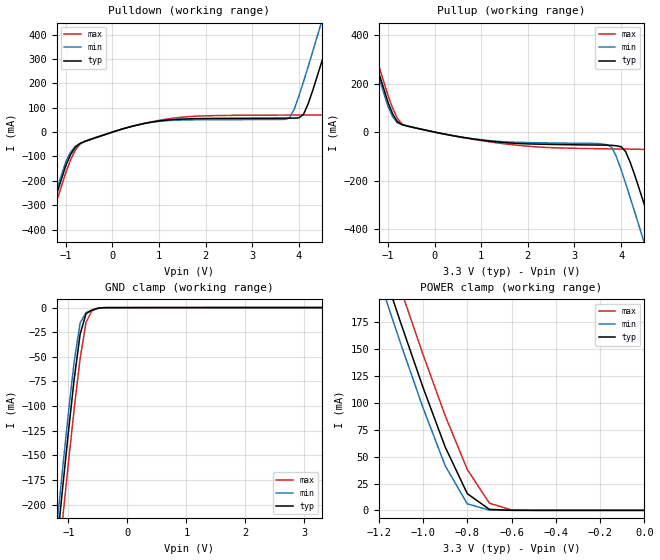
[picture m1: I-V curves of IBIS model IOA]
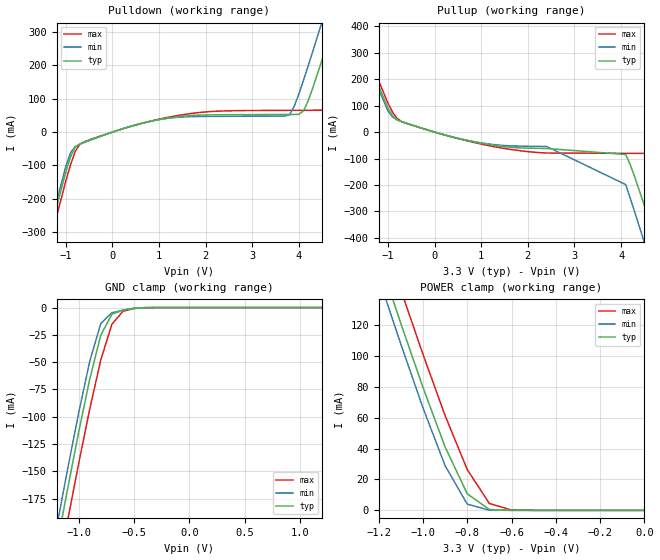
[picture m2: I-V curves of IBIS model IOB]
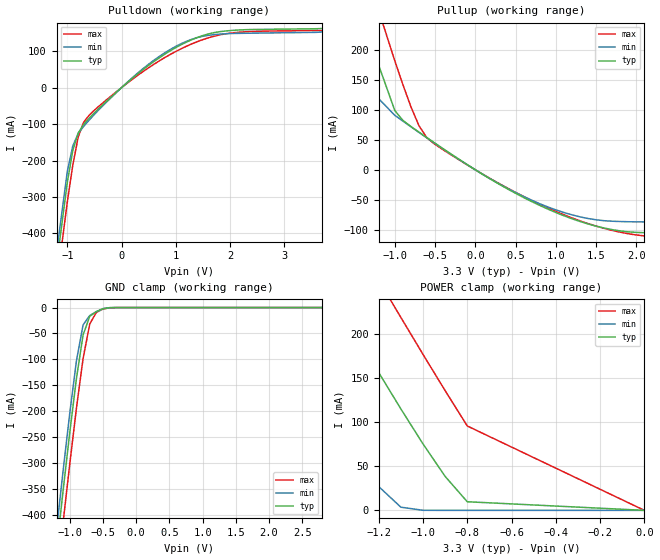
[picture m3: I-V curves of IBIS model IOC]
| IBIS file Qspan.ibs created by s2ibis2 version 2.1
[IBIS ver]   2.1
[File name]   qspn2a3.ibs
[File Rev]   1.0
[Date]   03- 03- 2000
[Notes]   The data is simulation based
|   This is for modelling purposes only.
|   History : #3591862.MI001.01 - Pin List corrections.
|   #3591862.MI001.02 - Revised Power Pins.
|   #3591862.MI001.03 - Updated with IDT formtting
|   This is the Qspan II (CA91L862A-XXE, 27mm PBGA) IBIS
|   MODEL for a 3.3 V PCI signalling environment.
[Disclaimer] This model is subject to change.
   Integrated Device Technology, Inc. ("IDT") hereby grants the
   user of this IBIS model a non-exclusive, nontransferable
   license to use this IBIS model under the following terms. The
   user is granted this license only to use the IBIS model and is
   not granted rights to sell, copy (except as needed to run the
   IBIS model), rent, lease or sub-license the IBIS model in
   whole or in part, or in modified form to anyone. The User may
   modify the IBIS model to suit its specific applications, but
   rights to derivative works and such modifications shall belong
   to IDT. This IBIS model is provided on an AS IS" basis and IDT
   makes absolutely no warranty with respect to the information
   contained herein. IDT DISCLAIMS AND CUSTOMER WAIVES ALL
   WARRANTIES, EXPRESS AND IMPLIED, INCLUDING WARRANTIES OF
   MERCHANTABILITY AND FITNESS FOR A PARTICULAR PURPOSE. THE
   ENTIRE RISK AS TO QUALITY AND PERFORMANCE IS WITH THE USER
   ACCORDINGLY, IN NO EVENT SHALL IDT BE LIABLE FOR ANY DIRECT OR
   INDIRECT DAMAGES, WHETHER IN CONTRACT OR TORT, INCLUDING ANY
   LOST PROFITS OR OTHER INCIDENTAL, CONSEQUENTIAL, EXEMPLARY, OR
   PUNITIVE DAMAGES ARISING OUT OF THE USE OR APPLICATION OF THE
   IBIS model. Further, IDT reserves the right to make changes
   without notice to any product herein to improve reliability,
   function, or design. IDT does not convey any license under
   patent rights or any other intellectual property rights,
   including those of third parties. IDT is not obligated to
   provide maintenance or support for the licensed IBIS model.
[Copyright]   Copyright 2009, Integrated Device Technology, Inc. all
   rights reserved.
|   Component QSPAN
[Component]   QSPAN
[Manufacturer]   Integrated Device Technology, Inc.
[Package]
| variable   typ   min   max
R_pkg   45m   22m   75m
L_pkg   2.5nH   1.1nH   4.3nH
C_pkg   1.3pF   1.2pF   1.4pF
[Pin]  signal_name   model_name
 A2   D26   IOA
 C2   D27   IOA
 B1   D28   IOA
 D3   D29   IOA
 C1   D30   IOA
 E4   D31   IOA
 E3   A26   IOA
 E1   A27   IOA
 F2   A28   IOA
 G2   A29   IOA
 H3   A30   IOA
 H2   A31   IOA
 G3   R/W   IOA
 H1   DSACK1/TA   IOB
 J4   DSACK0   IOB
 J3   SIZ1   IOA
 J2   SIZ0   IOA
 J1   SDA   IOB
 K3   SCL   OUTA
 L1   IMSEL   INA
 W19   VSS   GND
 L3   TMODE1   IOD
 M1   TMODE0   IOD
 M3   RESETI   INB
 N1   RESETO   IOF
 N3   BURST/TIP   IOA
 P2   TS   IOB
 R1   BB/BGACK   IOB
 R2   BR   OUTA
 T3   REQ   IOC
 T4   AD31   IOC
 V2   AD30   IOC
 U3   AD29   IOC
 W1   AD28   IOC
 W2   AD27   IOC
 T1   HALT/RETRY   IOB
 U2   GNT   IOC
 P4   RST   INC
 W11   PCLK   INC
 M20   BM_EN   IOD
 Y1   AD26   IOC
 Y2   AD25   IOC
 W3   AD24   IOC
 W4   C/BE3   IOC
 U5   AD23   IOC
 V7   AD22   IOC
 Y7   AD21   IOC
 V8   AD20   IOC
 W8   AD19   IOC
 Y8   AD18   IOC
 U9   AD17   IOC
 W9   AD16   IOC
 Y9   C/BE2   IOC
 W10   FRAME   IOC
 V10   IRDY   IOC
 Y10   TRDY   IOC
 Y11   DEVSEL   IOC
 V11   STOP   IOC
 U11   PERR   IOC
 Y12   PAR   IOC
 W12   C/BE1   IOC
 V12   AD15   IOC
 Y13   AD14   IOC
 W13   AD13   IOC
 V13   AD12   IOC
 Y14   AD11   IOC
 W14   AD10   IOC
 Y15   AD9   IOC
 V14   AD8   IOC
 W15   C/BE0   IOC
 Y16   IDSEL   INC
 U14   AD7   IOC
 W18   AD6   IOC
 V18   AD5   IOC
 Y20   AD4   IOC
 V19   AD3   IOC
 W20   AD2   IOC
 U18   AD1   IOC
 V20   AD0   IOC
 T19   CSREG   INA
 R20   CSPCI   INA
 P18   TC0   IOA
 P19   TC1   IOA
 P20   TC2   IOA
 N18   TC3   IOA
 N19   BERR/TEA   IOB
 N20   AS   IOB
 M17   BDIP   IOA
 M18   BG   INA
 J18   ENID   IOD
 K19   DACK/SDACK   INB
 K17   DONE   INA
 J19   QINT   IOE
 J17   DREQ   OUTA
 T18   INT   IOC
 U20   SERR   IOC
 G20   A0   IOA
 G19   A1   IOA
 F20   A2   IOA
 F19   A3   IOA
 E20   A4   IOA
 G17   A5   IOA
 F18   D0   IOA
 E19   D1   IOA
 E18   D2   IOA
 E17   D3   IOA
 C20   D4   IOA
 D18   D5   IOA
 P3   VSS   GND
 A10   QCLK   INA
 L20   VSS   GND
 A8   VSS   GND
 B20   D6   IOA
 B19   D7   IOA
 C18   D8   IOA
 A20   D9   IOA
 B18   D10   IOA
 A19   D11   IOA
 C17   A6   IOA
 B17   A7   IOA
 A18   A8   IOA
 B16   A9   IOA
 C16   A10   IOA
 C14   A11   IOA
 B14   A12   IOA
 A14   A13   IOA
 C13   A14   IOA
 B13   A15   IOA
 A13   DS   OUTA
 D12   D12   IOA
 C12   D13   IOA
 B12   D14   IOA
 B11   D15   IOA
 C11   D16   IOA
 A11   D17   IOA
 B10   D18   IOA
 C10   D19   IOA
 D10   A16   IOA
 A9   A17   IOA
 C9   A18   IOA
 D9   A19   IOA
 B8   A20   IOA
 C8   A21   IOA
 A7   A22   IOA
 B7   A23   IOA
 A6   A24   IOA
 C7   A25   IOA
 B6   D20   IOA
 D7   D21   IOA
 A3   D22   IOA
 C4   D23   IOA
 D5   D24   IOA
 B3   D25   IOA
 J20   TCK   INF
 L18   TDI   INF
 M19   TDO   OUTA
 K20   TMS   INF
 K18   TRST   INF
 K1   ENUM   IOF
 N2   HS_HEALTHY   IOD
 L2   HS_LED   IOF
 L4   HS_SWITCH   IOD
 M4   PCI_DIS   IOD
 M2   PME   IOF
 C5   DP3   IOA
 A4   DP2   IOA
 B5   DP1   IOA
 C6   DP0   IOA
 B4   PCI_ARB_EN   IOD
 B15   BIDIR_CTRL/Test1 ING
 D14   RAM_WE/TEST2   IOD
 C15   TMODE[2]/Test3 IOD
 V5   EXT_GNT[1]   OUTB
 W5   EXT_GNT[2]   OUTB
 Y5   EXT_GNT[3]   OUTB
 V6   EXT_GNT[4]   OUTB
 U7   EXT_GNT[5]   OUTB
 W6   EXT_GNT[6]   OUTB
 Y17   EXT_REQ[1]   IOC
 V16   EXT_REQ[2]   IOC
 W17   EXT_REQ[3]   IOC
 Y18   EXT_REQ[4]   IOC
 U16   EXT_REQ[5]   IOC
 V17   EXT_REQ[6]   IOC
 R3   VH   POWER
 D1   VSS   GND
 F1   VSS   GND
 D2   VDD   POWER
 U1   VSS   GND
 T2   VDD   POWER
 V1   VSS   GND
 V3   VDD   POWER
 W7   VSS   GND
 V9   VSS   GND
 U12   VDD   POWER
 Y19   VDD   POWER
 U19   VDD   POWER
 T17   VSS   GND
 H19   VSS   GND
 G18   VDD   POWER
 D20   VDD   POWER
 D19   VSS   GND
 C19   VDD   POWER
 D16   VDD   POWER
 A12   VSS   GND
 D6   VDD   POWER
 D11   VDD   POWER
 D15   VDD   POWER
 F4   VDD   POWER
 F17   VDD   POWER
 K4   VDD   POWER
 L17   VDD   POWER
 R4   VDD   POWER
 R17   VDD   POWER
 U6   VDD   POWER
 U10   VDD   POWER
 U15   VDD   POWER
 A5   VDD   POWER
 E2   VDD   POWER
 B2   VDD   POWER
 A1   VSS   GND
 D4   VSS   GND
 D8   VSS   GND
 D13   VSS   GND
 D17   VSS   GND
 H4   VSS   GND
 H17   VSS   GND
 N4   VSS   GND
 N17   VSS   GND
 U4   VSS   GND
 U8   VSS   GND
 U13   VSS   GND
 U17   VSS   GND
| Models and submodels in the file (14): IOA (I/O), IOB (I/O), IOC (I/O), IOD (I/O), IOE (I/O), IOF (I/O), INA (Input), INB (Input), INC (Input), IND (Input), INF (Input), ING (Input), OUTA (Output), OUTB (Output)
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|   Model IOA
[Model]   IOA
Model_type   I/O
Polarity   Non-Inverting
Vinl =   0.8000V
Vinh =   2.0000V
C_comp   5.00pF   5.00pF   5.00pF
[Voltage Range]   3.3000V   3.0000V   4.0000V
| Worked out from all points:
|   slope of the pulldown table from 0 to 0.495 V, typ, clamps not added: 18.2 ohm
|   slope of the pullup table from 0 to 0.495 V, typ, clamps not added: 27.2 ohm
|   GND clamp passes 1 mA (typ) near -0.52 V on its own axis
|   POWER clamp passes 1 mA (typ) near -0.70 V on its own axis
[Pulldown]
| voltage   I(typ)   I(min)   I(max)
-3.3V     -1.576A    -1.558A    -1.604A
-1.5V     -432.5mA   -413.1mA   -463.7mA
-1V       -137.3mA   -121.2mA   -166mA
-800mV    -62.87mA   -58.79mA   -74.96mA
-500mV    -31.87mA   -32.96mA   -30.93mA
1V        45.56mA    44.16mA    48.21mA
3.7V      57.2mA     52.22mA    69.71mA
4V        58.41mA    148mA      69.9mA
4.5V      294.4mA    461.1mA    70.42mA
4.7V      421.5mA    591.5mA    77.39mA
5.3V      814mA      988.5mA    402.9mA
6.6V      1.688A     1.867A     1.263A
[Pullup]
| voltage   I(typ)   I(min)   I(max)
-3.3V     1.609A     1.592A     1.638A
-1.7V     557.5mA    538.6mA    588mA
-1.5V     428.5mA    409.4mA    459.4mA
-1V       122.4mA    105.5mA    151.3mA
-700mV    30.44mA    30.51mA    33.57mA
1.3V      -39.66mA   -37.29mA   -43.6mA
3.8V      -54.6mA    -62.87mA   -69.47mA
4.1V      -81.22mA   -213.1mA   -70.13mA
4.5V      -300mA     -458.7mA   -71.63mA
4.7V      -422.9mA   -584.6mA   -86.04mA
5.3V      -800.7mA   -966.3mA   -409.6mA
6.6V      -1.632A    -1.801A    -1.229A
[GND_clamp]
| voltage   I(typ)   I(min)   I(max)
-3.3V     -1.575A    -1.558A    -1.603A
-1.2V     -245.1mA   -225.4mA   -276.9mA
-1.1V     -185.2mA   -165.4mA   -216.9mA
-1V       -127mA     -107.6mA   -158.4mA
-900mV    -72.3mA    -54.37mA   -102.3mA
-800mV    -26.9mA    -15.62mA   -51.61mA
-700mV    -6.214mA   -5.156mA   -14.97mA
-600mV    -2.552mA   -2.501mA   -3.238mA
-500mV    -695.8uA   -617.9uA   -852uA
-400mV    -107.6uA   -78.58uA   -172.5uA
3.3V      28.55pA    37.85pA    -1.579uA
[POWER_clamp]
| voltage   I(typ)   I(min)   I(max)
-3.3V     1.609A     1.591A     1.638A
-1.2V     236mA      216.5mA    267.2mA
-1.1V     174.3mA    154.8mA    205.5mA
-1V       114.6mA    95.56mA    145.3mA
-900mV    59.17mA    41.7mA     88.32mA
-800mV    15.58mA    6.074mA    38.1mA
-700mV    917.4uA    198.5uA    6.641mA
-600mV    41.48uA    8.933uA    391uA
0V        28.55pA    15.28pA    402.7pA
[Ramp]
| variable   typ   min   max
dV/dt_r   1.1938/1.0833n   1.0738/1.1037n   1.4781/1.0201n
dV/dt_f   1.3746/0.6576n   1.2583/0.6707n   1.6602/0.6545n
R_load = 50.0000
| End [Model] IOA
|   Model IOB
[Model]   IOB
Model_type   I/O
Polarity   Non-Inverting
Vinl =   0.8000V
Vinh =   2.0000V
C_comp   5.00pF   5.00pF   5.00pF
[Voltage Range]   3.3000V   3.0000V   4.0000V
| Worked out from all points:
|   slope of the pulldown table from 0 to 0.495 V, typ, clamps not added: 23.4 ohm
|   slope of the pullup table from 0 to 0.495 V, typ, clamps not added: 21.1 ohm
|   GND clamp passes 1 mA (typ) near -0.52 V on its own axis
|   POWER clamp passes 1 mA (typ) near -0.70 V on its own axis
[Pulldown]
| voltage   I(typ)   I(min)   I(max)
-3.3V     -1.412A    -1.395A    -1.438A
-1.5V     -386.4mA   -368.6mA   -415.1mA
-900mV    -74.1mA    -62.08mA   -98.15mA
-700mV    -35.4mA    -36.6mA    -36.59mA
-500mV    -24.52mA   -25.57mA   -23.57mA
1.3V      44.42mA    43.02mA    47.13mA
3.8V      52.72mA    51.97mA    65.13mA
4.1V      63.59mA    155.8mA    65.28mA
4.5V      217.2mA    331.9mA    65.51mA
4.7V      305.5mA    422.4mA    70.09mA
5.3V      577.8mA    698mA      295.9mA
6.6V      1.186A     1.309A     892.4mA
[Pullup]
| voltage   I(typ)   I(min)   I(max)
-3.3V     1.118A     1.106A     1.138A
-1.9V     478.2mA    465.2mA    499.2mA
-1.7V     388mA      374.9mA    409.2mA
-1V       89.64mA    79.2mA     108.7mA
-600mV    32.82mA    33.32mA    32.7mA
1V        -42.36mA   -40.74mA   -45.36mA
2.4V      -61.9mA    -54.17mA   -79.11mA
4.1V      -84.69mA   -198.5mA   -80.23mA
4.5V      -278mA     -416.8mA   -80.51mA
4.7V      -387.4mA   -528.9mA   -94.37mA
5.3V      -724.1mA   -869.2mA   -380.8mA
6.6V      -1.467A    -1.615A    -1.112A
[GND_clamp]
| voltage   I(typ)   I(min)   I(max)
-3.3V     -1.411A    -1.395A    -1.438A
-1.2V     -219.7mA   -201.6mA   -248.8mA
-1.1V     -166.1mA   -148mA     -195.1mA
-1V       -114.1mA   -96.4mA    -142.8mA
-900mV    -65.46mA   -49.1mA    -92.83mA
-800mV    -25.26mA   -14.59mA   -47.88mA
-700mV    -6.072mA   -4.689mA   -15.35mA
-600mV    -2.394mA   -2.36mA    -3.375mA
-500mV    -685.3uA   -610.9uA   -846.3uA
-400mV    -76.55uA   -48.08uA   -135.9uA
1.2V      4.332pA    -1.927pA   212.7pA
[POWER_clamp]
| voltage   I(typ)   I(min)   I(max)
-3.3V     1.117A     1.105A     1.137A
-1.2V     163.9mA    150.4mA    185.6mA
-1.1V     121mA      107.6mA    142.7mA
-1V       79.56mA    66.32mA    101mA
-900mV    41.02mA    28.91mA    61.3mA
-800mV    10.7mA     4.026mA    26.39mA
-700mV    530.2uA    85.3uA     4.443mA
-600mV    12.01uA    1.252uA    210.9uA
0V        46.55pA    30.21pA    403.7pA
[Ramp]
| variable   typ   min   max
dV/dt_r   1.3368/0.5001n   1.2090/0.4937n   1.6416/0.4419n
dV/dt_f   1.2654/0.2879n   1.1628/0.2678n   1.5276/0.2973n
R_load = 50.0000
| End [Model] IOB
|   Model IOC
[Model]   IOC
Model_type   I/O
Polarity   Non-Inverting
Vinl =   0.8000V
Vinh =   2.0000V
C_comp   5.00pF   5.00pF   5.00pF
[Voltage Range]   3.3000V   3.0000V   3.5000V
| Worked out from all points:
|   slope of the pulldown table from 0 to 0.495 V, typ, clamps not added: 8.19 ohm
|   slope of the pullup table from 0 to 0.495 V, typ, clamps not added: 12.7 ohm
|   GND clamp passes 1 mA (typ) near -0.44 V on its own axis
[Pulldown]
| voltage   I(typ)   I(min)   I(max)
-3.3V     -3.036A    -3.001A    -3.093A
-1.5V     -828mA     -790.5mA   -888.2mA
-1V       -258.8mA   -229mA     -312.4mA
-900mV    -172.7mA   -160.1mA   -212.7mA
-800mV    -124.4mA   -125.9mA   -135.4mA
-700mV    -100.9mA   -106.5mA   -95.31mA
-500mV    -69.01mA   -73.28mA   -61.83mA
200mV     25.72mA    27.27mA    22.91mA
1V        109.7mA    113mA      99.07mA
1.4V      137.5mA    137.3mA    126.1mA
2V        156.3mA    148.1mA    149.3mA
3.7V      162mA      152.5mA    156.5mA
[Pullup]
| voltage   I(typ)   I(min)   I(max)
-3.3V     1.071A     928.4mA    1.178A
-1.7V     372.7mA    236.2mA    478mA
-1.5V     287.7mA    160.6mA    391.8mA
-1V       98.94mA    90.94mA    181.9mA
-800mV    72.32mA    71.85mA    105.3mA
-700mV    62.91mA    62.44mA    73.61mA
-600mV    53.56mA    53.13mA    53.21mA
-500mV    44.32mA    43.94mA    42.33mA
300mV     -24.37mA   -23.78mA   -23.28mA
900mV     -65.6mA    -62.02mA   -63.68mA
1.5V      -94.12mA   -83.54mA   -94.04mA
2.1V      -105.1mA   -87.03mA   -110.5mA
[GND_clamp]
| voltage   I(typ)   I(min)   I(max)
-3.3V     -3.035A    -3A        -3.092A
-1.2V     -467.3mA   -428.9mA   -528.9mA
-1.1V     -351.9mA   -313.7mA   -413.4mA
-1V       -240.4mA   -203mA     -300.9mA
-900mV    -136.5mA   -102.5mA   -193.8mA
-800mV    -52.76mA   -33.41mA   -98.26mA
-700mV    -16.83mA   -15.35mA   -31.79mA
-600mV    -7.942mA   -7.882mA   -9.164mA
-500mV    -2.275mA   -1.992mA   -2.74mA
-300mV    -7.679uA   -2.34uA    -30.21uA
2.8V      217pA      169.4pA    822.9pA
[POWER_clamp]
| voltage   I(typ)   I(min)   I(max)
-3.3V     1.07A      926.7mA    1.177A
-1.8V     412.6mA    270.5mA    519.5mA
-1.7V     369.3mA    227.7mA    476.1mA
-1.5V     283.1mA    143.3mA    389.5mA
-1.4V     240.4mA    102.2mA    346.4mA
-1.3V     198mA      62.75mA    303.5mA
-1.2V     156.2mA    27mA       260.9mA
-1.1V     115mA      3.612mA    218.7mA
-1V       75.35mA    75.33uA    176.8mA
-900mV    38.5mA     1.103uA    135.7mA
-800mV    9.76mA     15.99nA    95.64mA
0V        246.5pA    181pA      1.468nA
[Ramp]
| variable   typ   min   max
dV/dt_r   1.5666/0.7294n   1.4148/0.7336n   1.6446/0.8117n
dV/dt_f   1.6987/0.8254n   1.5596/0.6190n   1.7612/1.1369n
R_load = 50.0000
| End [Model] IOC
